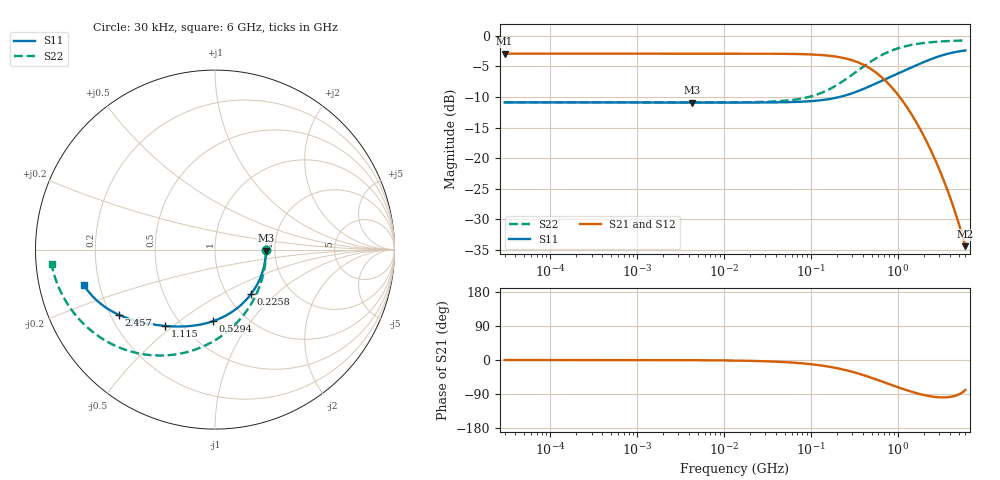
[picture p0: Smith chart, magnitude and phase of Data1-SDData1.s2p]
!EMIF06-MSD04F3
!Simulation
!24/03/11  09:16
!Start Freq. :30.000kHz; Stop Freq. : 6.000GHz
!Number of points : 1592; Sweep : LOGARITHMIC
!A2-A3 (Data1-SDData1)
!Freq ReS11 ImS11 ReS21 ImS21 ReS12 ImS12 ReS22 ImS22
# Hz  S  RI  R  50
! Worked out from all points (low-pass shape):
!   1592 points, 30 kHz to 6 GHz, reference 50 ohm
!   highest |S21| = -2.92 dB at 30 kHz (marker M1); lowest = -34.4 dB at 6 GHz (marker M2)
!   |S21| within 3 dB of the highest: start of sweep to 549.6 MHz
!   lowest |S11| = -10.9 dB at 4.27 MHz (marker M3), VSWR 1.79, Z = 89.7 - j1.04 ohm
!   |S11| at or under -10 dB: start of sweep to 215.5 MHz
!   |S22| runs from -10.9 to -0.8 dB; largest |S21 - S12| = 2e-15
!   S11 on the Smith chart (normalised r, x): 30 kHz: 1.80, -0.00; 225.8 MHz: 1.28, -0.71; 529.4 MHz: 0.71, -0.67; 1.115 GHz: 0.41, -0.47; 2.457 GHz: 0.23, -0.29; 6 GHz: 0.14, -0.13
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30000  0.2855 -0.000523  0.7142 -0.000312  0.7142 -0.000312  0.2857 -0.000211
231093.6  0.2844 -0.000788  0.7135 -0.0006  0.7135 -0.0006  0.2853 -0.000621
1766531  0.2841 -0.00232  0.7134 -0.00253  0.7134 -0.00253  0.2852 -0.00361
4270263  0.284 -0.00535  0.7133 -0.00597  0.7133 -0.00597  0.2852 -0.00864
1.350376e7  0.2837 -0.0167  0.7129 -0.0187  0.7129 -0.0187  0.2846 -0.0272
4.336319e7  0.2806 -0.0534  0.7088 -0.0598  0.7088 -0.0598  0.2788 -0.087
6.820056e7  0.2755 -0.0834  0.7021 -0.0933  0.7021 -0.0933  0.2694 -0.1358
1.032257e8  0.2647 -0.1243  0.6879 -0.1387  0.6879 -0.1387  0.2495 -0.202
1.586553e8  0.24 -0.1846  0.6557 -0.2043  0.6557 -0.2043  0.2043 -0.2981
2.258333e8  0.2004 -0.248  0.6043 -0.2707  0.6043 -0.2707  0.132 -0.3964
2.778356e8  0.1651 -0.289  0.5588 -0.3111  0.5588 -0.3111  0.0679 -0.4572
3.39199e8  0.1208 -0.3284  0.5024 -0.3466  0.5024 -0.3466  -0.0117 -0.5119
4.303164e8  0.0546 -0.3707  0.4197 -0.3778  0.4197 -0.3778  -0.129 -0.5631
5.294049e8  -0.0129 -0.3996  0.338 -0.389  0.338 -0.389  -0.2458 -0.5871
6.463304e8  -0.0833 -0.418  0.257 -0.3826  0.257 -0.3826  -0.3631 -0.5875
7.890804e8  -0.1554 -0.4271  0.1806 -0.3592  0.1806 -0.3592  -0.4761 -0.5655
1.114606e9  -0.2768 -0.4253  0.0753 -0.2893  0.0753 -0.2893  -0.6413 -0.4879
1.611095e9  -0.3996 -0.4069  0.0109 -0.1996  0.0109 -0.1996  -0.7628 -0.3812
2.45728e9  -0.5337 -0.3642  -0.0124 -0.1114  -0.0124 -0.1114  -0.8445 -0.2644
3.093532e9  -0.5997 -0.3285  -0.0117 -0.0762  -0.0117 -0.0762  -0.8715 -0.2087
3.835199e9  -0.653 -0.2884  -0.0073 -0.0515  -0.0073 -0.0515  -0.8892 -0.162
6e9  -0.7322 -0.1949  0.00364 -0.0188  0.00364 -0.0188  -0.9103 -0.0785
